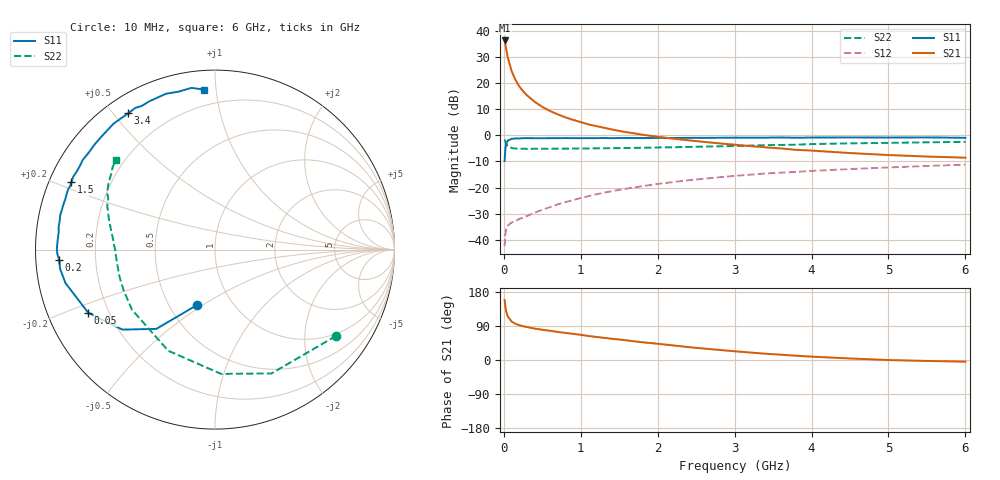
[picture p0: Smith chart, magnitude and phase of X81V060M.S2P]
! SIEMENS Small Signal Semiconductors
! BFP136W
! Si NPN RF Bipolar Junction Transistor in SOT343
! VCE = 1 V  IC = 60 mA
! Common Emitter S-Parameters:  September  1994
# GHz  S  MA  R  50
!  f  S11  S21  S12  S22
! GHz  MAG  ANG  MAG  ANG  MAG  ANG  MAG  ANG
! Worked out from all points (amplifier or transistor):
!   40 points, 10 MHz to 6 GHz, reference 50 ohm
!   highest |S21| = 36.2 dB at 10 MHz (marker M1)
!   |S21| within 3 dB of that: start of sweep to 28.77 MHz
!   unconditionally stable (mu >= 1): 512.9 MHz to 2.973 GHz; 3.114 GHz to 3.272 GHz; 3.738 GHz to 3.878 GHz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
!   at 200 MHz: K = 0.63, MSG = 25.3 dB, |S12| = -32.0 dB
!   at 1.5 GHz: K = 1.13, MAG = 9.1 dB, |S12| = -20.9 dB
!   at 6 GHz: K = 1.02, MAG = 0.4 dB, |S12| = -11.2 dB
!   S11 on the Smith chart (normalised r, x): 10 MHz: 0.69, -0.47; 50 MHz: 0.12, -0.23; 200 MHz: 0.07, -0.03; 1.5 GHz: 0.06, +0.22; 3.4 GHz: 0.07, +0.55; 6 GHz: 0.10, +0.93
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0.01  0.3236 -107.8  64.79 158.2  0.0076 66.4  0.8282 -35.5
0.02  0.5495 -126.5  54.31 140.9  0.0128 53.8  0.7583 -65.5
0.03  0.6822 -139.2  44.8 129.0  0.0159 44.8  0.6933 -87.2
0.05  0.7891 -153.5  31.26 115.3  0.0186 34.3  0.6209 -114.8
0.1  0.8538 -167.4  17 101.7  0.0215 29.7  0.5711 -144.2
0.15  0.8697 -172.9  11.51 95.6  0.023 33.3  0.5571 -155.9
0.2  0.8702 -176.2  8.613 91.8  0.0252 35.9  0.5534 -162.1
0.25  0.8791 -178.6  6.95 89.0  0.0267 38.7  0.5527 -166.0
0.3  0.8812 179.6  5.803 87.0  0.0286 41.3  0.5503 -168.8
0.4  0.8778 176.1  4.369 83.0  0.0331 46.8  0.5509 -172.3
0.5  0.8764 173.7  3.484 79.8  0.0378 49.8  0.5517 -174.8
0.6  0.8801 171.7  2.909 77.2  0.0423 53.0  0.5529 -176.4
0.7  0.8802 169.2  2.51 74.0  0.0478 55.1  0.5544 -177.6
0.9  0.8814 165.8  1.969 68.9  0.0577 57.4  0.5568 179.9
1.1  0.8802 161.3  1.613 63.3  0.0685 58.3  0.5605 178.3
1.5  0.8842 154.8  1.21 54.0  0.0904 58.2  0.5679 175.0
2.2  0.8871 142.5  0.862 38.5  0.1275 53.6  0.5896 169.3
3.2  0.8995 125.5  0.621 19.8  0.1761 44.2  0.6346 160.0
3.4  0.9 122.5  0.588 16.6  0.186 42.2  0.6473 158.1
4.5  0.9102 107.5  0.457 4.0  0.2261 31.9  0.7006 147.8
5.5  0.9106 98.3  0.392 -2.5  0.2589 23.9  0.7336 140.9
6  0.8938 94.0  0.373 -4.4  0.275 19.5  0.746 137.8
